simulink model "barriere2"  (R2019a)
settings: Solver=ode45  StartTime=0.0  StopTime=2  RelTol=1e-3  EnableMultiTasking=on

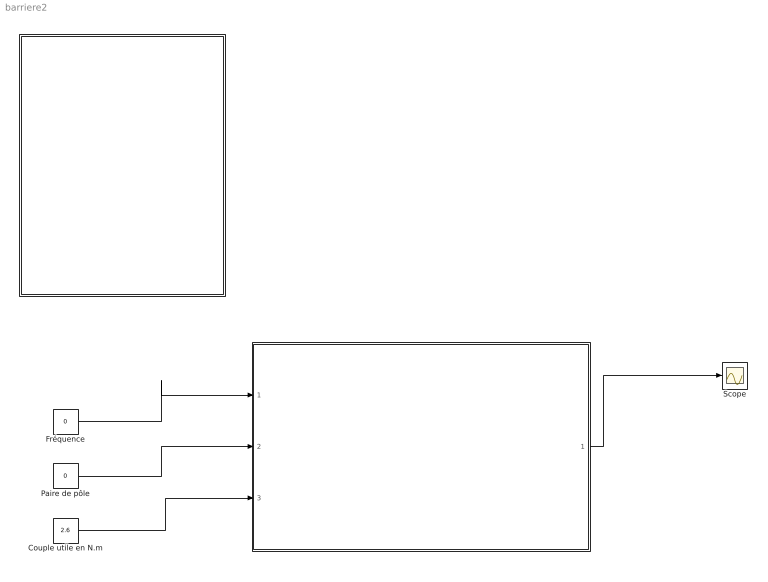
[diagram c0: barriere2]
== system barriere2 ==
  "  " : Subsystem
  "    " : Subsystem
  Couple utile en N.m : Constant  Value=2.6
  Fréquence : Constant  Value=0
  Paire de pôle : Constant  Value=0
  Scope : Scope
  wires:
  "  "/1(Out1) -> Scope/1
  Fréquence/1 -> "  "/1(In1)
  Paire de pôle/1 -> "  "/2(In2)
  Couple utile en N.m/1 -> "  "/3(In3)

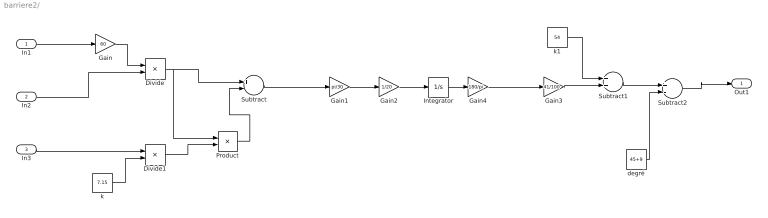
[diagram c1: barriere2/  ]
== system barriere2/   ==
  In1 : Inport
  In2 : Inport  Port=2
  In3 : Inport  Port=3
  Divide : Product  Inputs=*/
  Divide1 : Product  Inputs=*/
  Gain : Gain  Gain=60
  Gain1 : Gain  Gain=pi/30
  Gain2 : Gain  Gain=1/20
  Gain3 : Gain  Gain=41/100
  Gain4 : Gain  Gain=180/pi
  Integrator : Integrator
  Product : Product
  Subtract : Sum  Inputs=+-
  Subtract1 : Sum
  Subtract2 : Sum  Inputs=+-
  degré : Constant  Value=45+9
  k : Constant  Value=7.15
  k1 : Constant  Value=54
  Out1 : Outport
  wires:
  In1/1 -> Gain/1
  Gain/1 -> Divide/1
  In2/1 -> Divide/2
  In3/1 -> Divide1/1
  k/1 -> Divide1/2
  Divide/1 -> Product/1, Subtract/1
  Divide1/1 -> Product/2
  Product/1 -> Subtract/2
  Subtract/1 -> Gain1/1
  k1/1 -> Subtract1/1
  Gain2/1 -> Integrator/1
  Gain3/1 -> Subtract1/2
  Gain1/1 -> Gain2/1
  Gain4/1 -> Gain3/1
  Integrator/1 -> Gain4/1
  Subtract1/1 -> Subtract2/1
  Subtract2/1 -> Out1/1
  degré/1 -> Subtract2/2

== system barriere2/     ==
